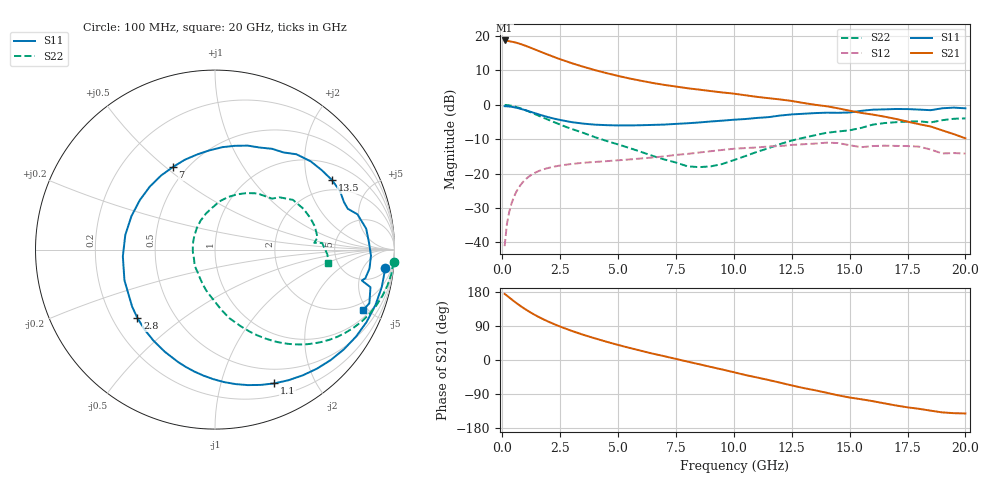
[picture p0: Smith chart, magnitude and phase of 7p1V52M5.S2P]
! Infineon Technologies  Discrete & RF Semiconductors
! bfp620
! VCE =  1.5 V,  IC =  2.5 mA
! Common Emitter S-Parameters:  Sep 2002
# GHz  S  MA  R  50
!  f  S11  S21  S12  S22
! GHz  MAG  ANG  MAG  ANG  MAG  ANG  MAG  ANG
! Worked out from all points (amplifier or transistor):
!   59 points, 100 MHz to 20 GHz, reference 50 ohm
!   highest |S21| = 18.7 dB at 100 MHz (marker M1)
!   |S21| within 3 dB of that: start of sweep to 1.548 GHz
!   unconditionally stable (mu >= 1): 5.592 GHz to 13.24 GHz; 14.25 GHz to 15.64 GHz; 17.37 GHz to end of sweep
!   at 1 GHz: K = 0.19, MSG = 19.4 dB, |S12| = -21.7 dB
!   at 5.5 GHz: K = 0.99, MSG = 11.8 dB, |S12| = -15.9 dB
!   at 20 GHz: K = 1.44, MAG = -1.7 dB, |S12| = -14.2 dB
!   S11 on the Smith chart (normalised r, x): 100 MHz: 7, -16; 1.1 GHz: 0.33, -1.48; 2.8 GHz: 0.30, -0.35; 7 GHz: 0.42, +0.53; 13.5 GHz: 1.56, +2.85; 20 GHz: 1.43, -4.65
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0.1  0.9546 -6.1  8.634 174.5  0.0088 82.0  0.9974 -4.0
0.3  0.9459 -19.1  8.422 165.0  0.0278 79.8  0.9817 -11.7
0.6  0.9081 -37.7  8.001 150.7  0.054 68.9  0.9313 -22.8
0.8  0.8731 -49.5  7.64 141.9  0.0691 62.0  0.8864 -29.4
1.1  0.8153 -66.1  7.022 130.0  0.0879 52.7  0.8112 -38.3
1.3  0.7768 -76.4  6.603 122.7  0.0979 47.3  0.7603 -43.4
1.5  0.7398 -86.1  6.204 115.9  0.1062 42.6  0.7113 -48.0
1.9  0.6739 -103.9  5.489 103.8  0.1186 34.6  0.6235 -55.8
2.4  0.6124 -124.0  4.735 90.6  0.1293 26.9  0.5322 -63.8
2.8  0.5762 -138.6  4.257 81.4  0.1353 21.9  0.4709 -69.4
3.5  0.5327 -161.3  3.58 66.5  0.1437 14.8  0.3909 -78.1
4  0.5148 -175.8  3.199 57.1  0.1476 10.6  0.3388 -83.8
5  0.5015 158.1  2.634 39.7  0.1561 4.5  0.2656 -94.5
6  0.5052 136.0  2.238 24.2  0.1659 -0.8  0.2066 -109.0
7  0.5164 116.9  1.949 10.0  0.1782 -5.5  0.1602 -126.8
9  0.5721 85.9  1.585 -18.2  0.2115 -18.1  0.1273 165.8
10.5  0.6216 66.1  1.377 -39.7  0.235 -30.9  0.18 116.5
12  0.6986 49.5  1.197 -59.8  0.2516 -42.6  0.2692 84.8
13.5  0.758 30.8  1.003 -79.8  0.2731 -56.5  0.3611 60.7
15  0.7739 17.1  0.821 -99.0  0.2585 -76.1  0.4263 41.8
17  0.8697 -2.2  0.624 -120.0  0.2527 -87.7  0.5592 18.5
20  0.8901 -22.3  0.326 -141.1  0.1957 -107.0  0.6351 -6.6
